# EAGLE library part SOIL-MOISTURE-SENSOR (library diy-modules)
Soil Moisture Sensor Click here to find device on ebay.com
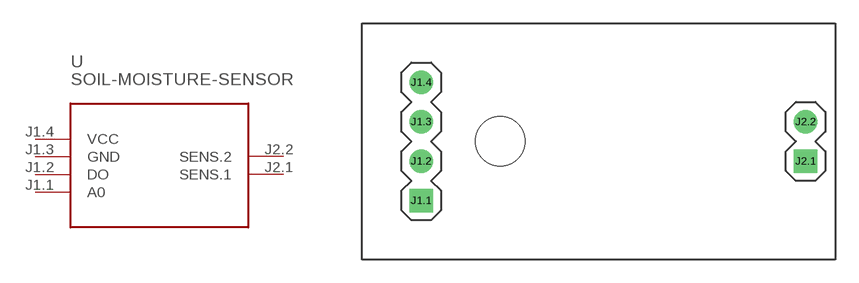
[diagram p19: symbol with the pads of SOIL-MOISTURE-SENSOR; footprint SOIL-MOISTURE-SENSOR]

Designator prefix -

## SOIL-MOISTURE-SENSOR  [SOIL-MOISTURE-SENSOR]
J1.1  A0
J1.2  DO  out
J1.3  GND  pwr
J1.4  VCC  pwr
J2.1  SENS.1
J2.2  SENS.2

## Footprint SOIL-MOISTURE-SENSOR (pad centres in mm)
Soil Moisture Sensor
drill 1 square: J1.1 -11.43,-3.81; J2.1 13.335,-1.27
drill 1: J1.2 -11.43,-1.27; J1.3 -11.43,1.27; J1.4 -11.43,3.81; J2.2 13.335,1.27
hole 3.2 at -6.35,0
